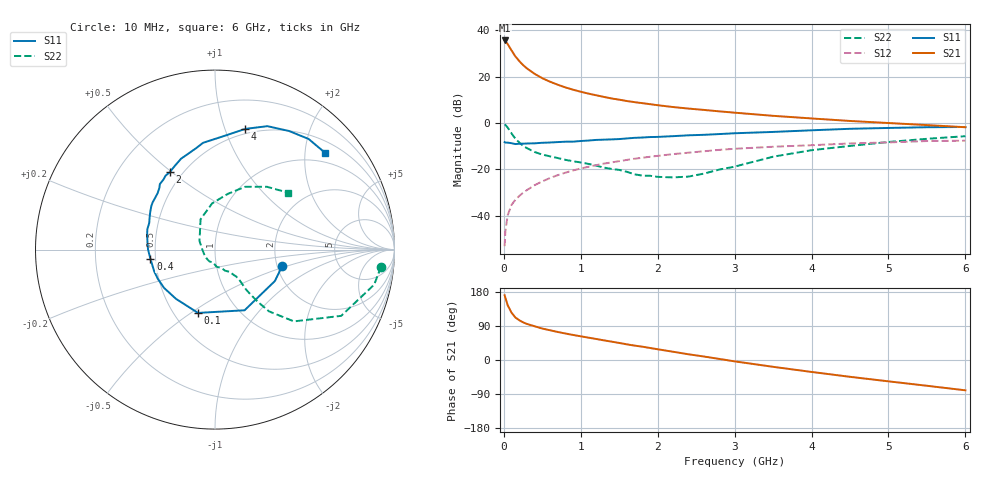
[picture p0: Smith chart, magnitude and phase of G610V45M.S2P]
! SIEMENS Small Signal Semiconductors
! BFG193
! Si NPN RF Bipolar Junction Transistor in SOT223
! VCE = 10 V  IC = 45 mA
! Common Emitter S-Parameters:  August  1996
# GHz  S  MA  R  50
!  f  S11  S21  S12  S22
! GHz  MAG  ANG  MAG  ANG  MAG  ANG  MAG  ANG
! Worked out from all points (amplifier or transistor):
!   36 points, 10 MHz to 6 GHz, reference 50 ohm
!   highest |S21| = 35.6 dB at 10 MHz (marker M1)
!   |S21| within 3 dB of that: start of sweep to 76.3 MHz
!   unconditionally stable (mu >= 1): 539.1 MHz to 2.502 GHz
!   at 250 MHz: K = 0.87, MSG = 27.5 dB, |S12| = -30.1 dB
!   at 1.4 GHz: K = 1.04, MAG = 12.5 dB, |S12| = -17.0 dB
!   at 6 GHz: K = 0.89, MSG = 2.9 dB, |S12| = -7.7 dB
!   S11 on the Smith chart (normalised r, x): 10 MHz: 2.13, -0.46; 100 MHz: 0.66, -0.53; 400 MHz: 0.47, -0.06; 2 GHz: 0.43, +0.49; 4 GHz: 0.45, +1.18; 6 GHz: 0.76, +2.46
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0.01  0.3856 -13.7  60.01 170.9  0.0022 85.7  0.9298 -5.9
0.02  0.3768 -27.7  58.27 164.3  0.0047 77.5  0.9083 -12.4
0.05  0.3761 -64.0  50.17 144.6  0.0102 70.0  0.794 -27.7
0.1  0.3652 -105.0  36.57 124.9  0.0171 66.1  0.5943 -42.3
0.15  0.3501 -128.3  27.17 112.2  0.022 64.0  0.4575 -48.8
0.2  0.3551 -143.0  21.6 105.0  0.0265 65.3  0.3787 -50.6
0.25  0.3577 -152.8  17.7 99.4  0.0313 66.0  0.3199 -51.6
0.3  0.3599 -160.1  14.98 95.2  0.0356 67.1  0.2857 -52.1
0.4  0.3633 -171.7  11.44 89.0  0.0454 67.5  0.2362 -51.5
0.5  0.3732 179.8  9.204 83.0  0.0549 66.9  0.2076 -51.1
0.6  0.3782 174.0  7.737 78.5  0.0649 66.2  0.1904 -51.8
0.7  0.3863 168.1  6.669 74.0  0.0747 65.1  0.175 -53.7
0.9  0.3951 158.1  5.205 66.1  0.0946 61.5  0.149 -56.3
1.1  0.4172 149.9  4.285 59.0  0.1132 58.6  0.1307 -64.2
1.6  0.4631 132.0  2.965 41.3  0.1595 48.0  0.0883 -88.6
2  0.4994 120.4  2.41 28.3  0.195 39.1  0.0687 -129.4
2.2  0.5184 115.4  2.2 21.8  0.2124 34.7  0.0669 -147.7
3.5  0.6394 84.5  1.423 -18.0  0.3065 3.9  0.187 115.5
4  0.6934 75.9  1.249 -31.5  0.3305 -5.8  0.2582 93.5
4.5  0.7471 67.0  1.102 -44.4  0.3611 -15.9  0.3189 77.0
5.5  0.8074 49.8  0.898 -68.0  0.4067 -39.0  0.4543 50.4
6  0.817 41.2  0.808 -80.0  0.4138 -52.4  0.5174 37.7
